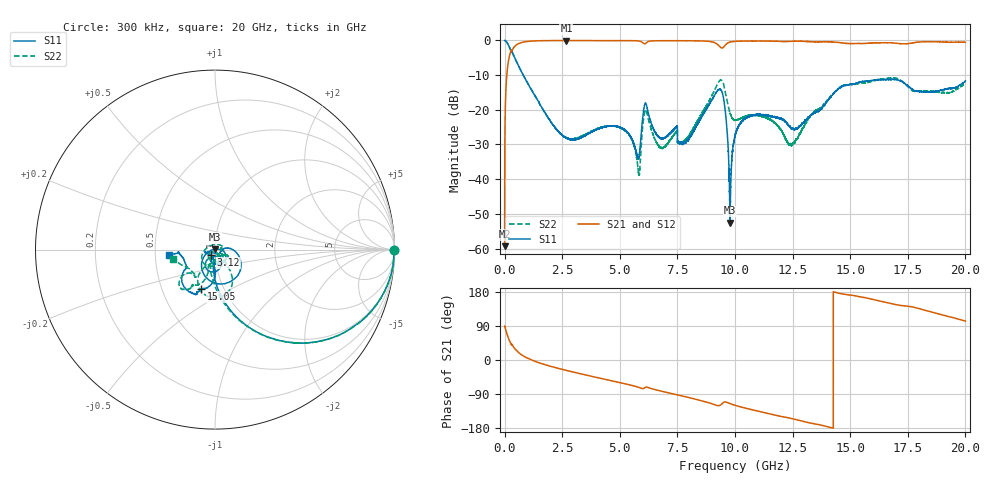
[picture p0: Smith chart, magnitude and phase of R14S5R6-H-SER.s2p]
!{R14S5R6}
!Johanson Technology Inc.
!www.johansontechnology.com
!Test Board Conditions:
!Substrate Type  RO4350B
!Substrate Thickness  20 mil
!Substrate Dk  3.66
!TL Type: GCPW
!TL Trace Width  36 mil
!TL Gap  12 mil
!Electrode orientation  Horizontal
!DUT TOPOLOGY	SERIES
!Mounting Pad LxW  26x36 mil
! Created Wed Nov 25 17:33:21 2020
! 2 Port Network Data from SP1.SP block
! freq  magS11  angS11  magS21  angS21  magS12  angS12  magS22  angS22
# khz S ma R 50
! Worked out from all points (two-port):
!   20001 points, 300 kHz to 20 GHz, reference 50 ohm
!   highest |S21| = -0.02 dB at 2.682 GHz (marker M1); lowest = -59.3 dB at 300 kHz (marker M2)
!   |S21| within 3 dB of the highest: 281.9 MHz to 300 MHz (18.04 MHz wide, 6.2 % of centre); 309.6 MHz to end of sweep
!   lowest |S11| = -52.6 dB at 9.784 GHz (marker M3), VSWR 1.00, Z = 50 + j0.232 ohm
!   |S11| at or under -10 dB: 809.4 MHz to end of sweep
!   |S22| runs from -38.9 to 0.0 dB; largest |S21 - S12| = 0.018
!   S11 on the Smith chart (normalised r, x): 300 kHz: open; 3.12 GHz: 0.95, -0.06; 15.05 GHz: 0.78, -0.36; 20 GHz: 0.59, -0.03
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300  0.9956 -0.2  0.001081 88.7  0.001026 92.0  0.9952 -0.2
110300  0.9306 -22.5  0.3623 67.4  0.3634 67.3  0.9305 -22.4
294300  0.6853 -49.3  0.722 40.3  0.7219 40.3  0.6861 -49.3
953300  0.258 -82.7  0.9638 6.1  0.9635 6.0  0.2589 -84.5
2682300  0.03922 -108.1  0.9977 -27.5  0.9965 -27.4  0.03966 -124.4
3120300  0.03778 -126.4  0.9963 -33.8  0.9964 -33.8  0.03877 -119.6
3334300  0.03991 -135.7  0.9959 -36.9  0.9958 -36.9  0.04135 -116.7
5061300  0.05494 -164.7  0.9943 -60.5  0.9937 -60.6  0.05423 -133.3
5809300  0.02009 -102.2  0.984 -72.0  0.9837 -71.9  0.013 -124.4
6137300  0.1226 -107.5  0.9148 -71.4  0.9153 -71.5  0.09952 -128.2
6667300  0.0414 -102.5  0.9916 -80.3  0.9905 -80.3  0.03084 130.0
7900300  0.03527 -9.5  0.9895 -97.7  0.9888 -97.7  0.0377 -19.8
9349300  0.1977 -70.2  0.8083 -119.5  0.8094 -119.6  0.2658 -83.5
9558300  0.1092 -133.2  0.841 -110.5  0.8447 -110.6  0.1966 -119.3
9784300  0.002354 99.7  0.9468 -115.0  0.9467 -114.9  0.09009 -111.7
1.00003e7  0.04169 -7.1  0.9696 -119.5  0.9699 -119.5  0.07063 -82.0
1.08693e7  0.08419 -58.5  0.9826 -133.1  0.981 -133.1  0.08343 -32.7
1.24183e7  0.05505 -109.7  0.973 -154.1  0.9731 -154.0  0.0314 -51.1
1.33343e7  0.08601 -92.9  0.9587 -167.1  0.9595 -167.1  0.08604 -106.2
1.50473e7  0.233 -109.6  0.903 171.0  0.8997 170.6  0.2327 -122.4
1.66673e7  0.2706 -118.6  0.9254 150.3  0.9188 150.1  0.2875 -129.4
2e7  0.2594 -173.9  0.941 102.8  0.9395 103.0  0.2414 -167.1
